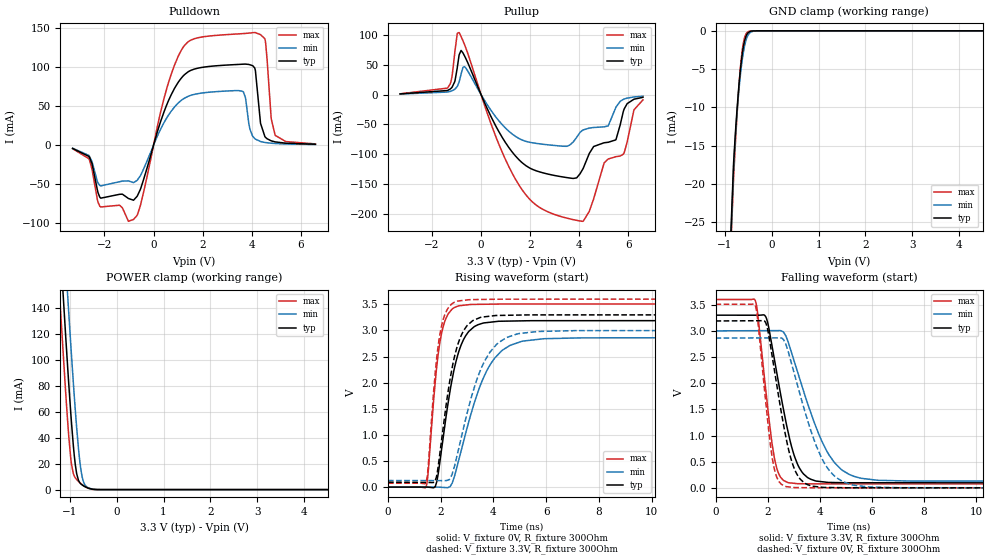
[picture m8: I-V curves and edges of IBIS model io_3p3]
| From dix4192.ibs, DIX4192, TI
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|   io_3p3 Model
[Model]   io_3p3
Model_type   3-state
Polarity   Non-Inverting
Vmeas = 1.65
Vref = 0
Cref = 2pF
Rref = 100000
|   typ   min   max
C_comp   31.7427pF   25.9206pF   37.4662pF
|C_comp_pullup   32.184pF   26.2805pF   37.987pF
|C_comp_pulldown   32.4791pF   26.6449pF   38.1628pF
| Where nom  PVT is Nominal Process, 3.3V, 27C
|   Fast PVT is Strong Process,  3.6V, -40C
|   Slow PVT is Weak Process,   3.0V, 105C
[Voltage Range]   3.3   3   3.6
[Temperature Range]   27   105   -40
[Pullup Reference]   3.3   3   3.6
[Pulldown Reference]   0   0   0
[Power Clamp Reference]   3.3   3   3.6
[GND Clamp Reference]   0   0   0
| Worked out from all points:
|   slope of the pulldown table from 0 to 0.495 V, typ, clamps not added: 10.2 ohm
|   slope of the pullup table from 0 to 0.495 V, typ, clamps not added: 11.2 ohm
|   GND clamp passes 1 mA (typ) near -0.56 V on its own axis
|   POWER clamp passes 1 mA (typ) near -0.59 V on its own axis
|   falling waveform, V_fixture 3.3V, R_fixture 300Ohm: 20-80 % time 761ps typ, 1.26ns min, 478ps max; typ from 3.3 V to 0.095 V
|   rising waveform, V_fixture 0V, R_fixture 300Ohm: 20-80 % time 649ps typ, 1.1ns min, 394ps max; typ from 0 V to 3.19 V
|   rising waveform, V_fixture 3.3V, R_fixture 300Ohm: 20-80 % time 614ps typ, 1.01ns min, 378ps max; typ from 0.095 V to 3.3 V
|   falling waveform, V_fixture 0V, R_fixture 300Ohm: 20-80 % time 689ps typ, 1.11ns min, 440ps max; typ from 3.19 V to 0 V
[Pulldown]
|   Voltage   I(typ)   I(min)   I(max)
-3.3V     -4.185mA   -3.787mA   -4.454mA
-2.637V   -14.34mA   -13.1mA    -17.26mA
-2.191V   -66.68mA   -51.62mA   -78.27mA
-815.1mV  -70.61mA   -48mA      -95.26mA
1.195V    88.4mA     59mA       125.1mA
3.65V     104mA      68.73mA    143.3mA
4.125V    99.15mA    8.551mA    144.6mA
4.363V    28.11mA    4.749mA    142mA
4.551V    10.64mA    3.483mA    135.2mA
4.798V    5.618mA    2.568mA    34.1mA
4.957V    4.292mA    2.196mA    13.05mA
6.6V      1.224mA    869.1uA    1.663mA
[GND Clamp]
|   Voltage   I(typ)   I(min)   I(max)
-3.3V     -1.052A    -978.4mA   -1.121A
-1.003V   -46.85mA   -48.77mA   -48.16mA
-815.1mV  -17.3mA    -17.98mA   -19.31mA
-765.6mV  -12.4mA    -12.84mA   -13.54mA
-716.1mV  -8.26mA    -8.79mA    -8.564mA
-676.5mV  -5.518mA   -6.188mA   -5.319mA
-636.9mV  -3.351mA   -4.098mA   -2.883mA
-577.5mV  -1.26mA    -1.896mA   -834.3uA
-528mV    -443.2uA   -845.6uA   -222.7uA
-478.5mV  -130.9uA   -327.2uA   -47.39uA
-260.7mV  0A         -1.313uA   0A
6.6V      0A         0A         0A
[Pullup]
|   Voltage   I(typ)   I(min)   I(max)
-3.3V     1.193mA    955.2uA    1.362mA
-1.36V    7.072mA    4.404mA    11.4mA
-894.3mV  66.92mA    21.2mA     104.3mA
-646.8mV  62.78mA    45.89mA    81.1mA
1.601V    -111.6mA   -74.87mA   -155.5mA
3.501V    -139.4mA   -86.76mA   -207.6mA
4.125V    -126.7mA   -60.28mA   -212.9mA
5.016V    -80.87mA   -54.12mA   -114.9mA
5.501V    -75.45mA   -21.02mA   -104.2mA
5.828V    -24.91mA   -7.527mA   -98.17mA
6.234V    -7.69mA    -3.897mA   -25.54mA
6.6V      -4.553mA   -2.682mA   -8.874mA
[POWER Clamp]
|   Voltage   I(typ)   I(min)   I(max)
-3.3V     1.547A     1.6A       1.506A
-1.261V   221.8mA    278.9mA    176.5mA
-1.201V   185.4mA    242.4mA    140.3mA
-1.181V   173.4mA    230.3mA    128.4mA
-1.092V   120.7mA    176.8mA    76.94mA
-1.063V   103.7mA    159.3mA    60.97mA
-1.033V   87.14mA    142.1mA    46.08mA
-963.6mV  51.24mA    103.1mA    19.41mA
-854.7mV  12.41mA    48.08mA    7.805mA
-745.8mV  3.823mA    11.52mA    4.15mA
-607.2mV  1.171mA    1.445mA    1.051mA
6.6V      0A         0A         0A
[Ramp]
R_load = 300
|   typ   min   max
dV/dt_r   1.91352/6.48966e-10   1.71722/1.10013e-09   2.10458/3.92641e-10
dV/dt_f   1.92296/7.59547e-10   1.72387/1.25598e-09   2.11532/4.77619e-10
[Falling Waveform]
V_fixture = 3.3V
V_fixture_min = 3V
V_fixture_max = 3.6V
R_fixture = 300Ohm
C_fixture = 0F
|   Time   V(typ)   V(min)   V(max)
0s        3.3V       3V         3.6V
1.526ns   3.3V       3.003V     3.578V
1.932ns   3.265V     3.004V     1.851V
2.249ns   2.485V     3.005V     598.4mV
2.467ns   1.871V     3.005V     226.1mV
2.778ns   1.084V     2.802V     101.6mV
3.311ns   306.4mV    1.956V     79.12mV
4.241ns   108.6mV    729.2mV    75.59mV
5.527ns   96.68mV    190mV      75.52mV
25ns      95.07mV    126.9mV    74.47mV
[Rising Waveform]
V_fixture = 0V
V_fixture_min = 0V
V_fixture_max = 0V
R_fixture = 300Ohm
C_fixture = 0F
|   Time   V(typ)   V(min)   V(max)
0s        -5.526nV   356nV      -33.67nV
1.442ns   280.5uV    138.9uV    3.681mV
1.794ns   10.82mV    172.6uV    2.022V
1.993ns   576.9mV    -1.816mV   2.843V
2.354ns   1.841V     7.946mV    3.362V
2.667ns   2.566V     486.7mV    3.469V
3.072ns   2.985V     1.265V     3.494V
3.759ns   3.151V     2.241V     3.502V
5.125ns   3.184V     2.797V     3.506V
25ns      3.189V     2.862V     3.508V
[Rising Waveform]
V_fixture = 3.3V
V_fixture_min = 3V
V_fixture_max = 3.6V
R_fixture = 300Ohm
C_fixture = 0F
|   Time   V(typ)   V(min)   V(max)
0s        95.07mV    126.9mV    74.47mV
1.442ns   89.31mV    125.3mV    85.57mV
1.778ns   106.4mV    124.9mV    2.109V
1.963ns   626.7mV    124.7mV    2.91V
2.327ns   1.981V     144.4mV    3.461V
2.631ns   2.703V     628.9mV    3.561V
3.009ns   3.097V     1.43V      3.585V
3.665ns   3.262V     2.413V     3.594V
4.94ns    3.294V     2.937V     3.599V
25ns      3.3V       3V         3.6V
[Falling Waveform]
|Gnd
V_fixture = 0V
V_fixture_min = 0V
V_fixture_max = 0V
R_fixture = 300Ohm
C_fixture = 0F
|   Time   V(typ)   V(min)   V(max)
0s        3.189V     2.862V     3.508V
1.526ns   3.194V     2.865V     3.484V
1.932ns   3.149V     2.866V     1.614V
2.19ns    2.465V     2.866V     533mV
2.403ns   1.803V     2.867V     146.4mV
2.694ns   985.7mV    2.752V     26.29mV
3.216ns   188.2mV    1.833V     4.863mV
4.049ns   13.56mV    593.2mV    1.128mV
5.237ns   1.44mV     58.38mV    1.064mV
25ns      22.94nV    891.3nV    -41.4nV
